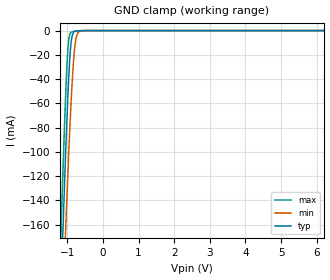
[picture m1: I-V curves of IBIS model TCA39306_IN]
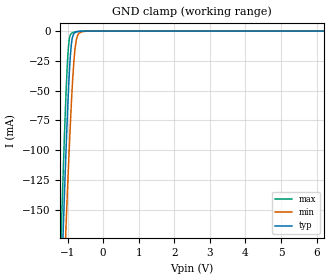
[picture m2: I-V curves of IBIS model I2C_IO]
|Texas Instruments Incorporated
| Low voltage FM+ I2C bus and SMBus voltage translator
| TCA39306
| Voltage Range : 0.9V-5.5V
| Package-type: DCU / DCT / DTM
| #pins/pkg drawing : 8-pin DCU /  8-pin DCT / 8-pin DTM
[IBIS Ver] 4.1
[File name] tca39306_5p0.ibs
[File Rev] 1.0
[Date] 07/01/2021
[Source]
| Texas Instruments Incorporated.
| 12500 TI Blvd
| Dallas, TX -75243
[Notes] Revision History:
| Rev 1.0: 07/01/2021
| - Initial version of the model
| - Model generated from simulations in SPECTRE
| - C_comp although listed in numerical order of value are
| obtained from varying PVT conditions. For PVT conditions for
| each specific value refer the buffer description under
| respective [Model]. IBIS model user is responsible for using
| appropriate C_comp to simulate for Signal Integrity.
| - Warnings regarding combined Non-monotonicity of various models have been
| reviewed and considered minor and can be ignored.
[Disclaimer]
| This model is designed as an aid for customers of Texas Instruments.
| TI and its licensors and suppliers make no warranties, either expressed
| or implied, with respect to this model, including the warranties of
| merchantability or fitness for a particular purpose. The model is
| provided solely on an "as is" basis. The entire risk as to its quality
| and performance is with the customer.
| This model is subject to change without notice. Texas Instruments
| Incorporated is not responsible for updating this model.
[Copyright]
(C) Copyright 2019 Texas Instruments Incorporated. All rights reserved.
| Component1 TCA39306DCU 8-PIN TSSOP
[Component] TCA39306_DCU
[Manufacturer] Texas Instruments Incorporated
[Package] |DCU 8-pin TSSOP
| variable typ   min   max
R_pkg 1.400e-02   1.300e-02   1.500e-02
L_pkg 1.289e-09   1.025e-09   2.014e-09
C_pkg 1.360e-13   6.600e-14   2.940e-13
[Pin]   signal_name   model_name   R_pin   L_pin   C_pin
1   GND   GND   1.400e-02   1.387e-09   1.760e-13
2   VREF1   I2C_IO   1.300e-02   1.026e-09   6.600e-14
3   SCL1   I2C_IO   1.300e-02   1.032e-09   6.700e-14
4   SDA1   I2C_IO   1.500e-02   2.014e-09   2.940e-13
5   SDA2   I2C_IO   1.400e-02   1.412e-09   1.780e-13
6   SCL2   I2C_IO   1.300e-02   1.030e-09   6.600e-14
7   VREF2   I2C_IO   1.300e-02   1.025e-09   6.600e-14
8   EN   TCA39306_IN   1.400e-02   1.386e-09   1.760e-13
[Series Pin Mapping]   pin_2   model_name   function_table_group
2   7   I2C_IO_S   1
3   6   I2C_IO_S   1
4   5   I2C_IO_S   1
[Series Switch Groups]
| Function Group States
On  1 /
Off 1 /
| Component2 TCA39306DCT 8-PIN TSSOP
[Component] TCA39306_DCT
[Manufacturer] Texas Instruments Incorporated
[Package] |DCU 8-pin TSSOP
| variable typ   min   max
R_pkg   2.900e-02   2.800e-02   3.100e-02
L_pkg   1.796e-09   1.666e-09   1.924e-09
C_pkg   1.090e-13   8.300e-14   1.360e-13
[Pin]   signal_name   model_name   R_pin   L_pin   C_pin
1   GND   GND   1.400e-02   1.387e-09   1.760e-13
2   VREF1   I2C_IO   1.300e-02   1.026e-09   6.600e-14
3   SCL1   I2C_IO   1.300e-02   1.032e-09   6.700e-14
4   SDA1   I2C_IO   1.500e-02   2.014e-09   2.940e-13
5   SDA2   I2C_IO   1.400e-02   1.412e-09   1.780e-13
6   SCL2   I2C_IO   1.300e-02   1.030e-09   6.600e-14
7   VREF2   I2C_IO   1.300e-02   1.025e-09   6.600e-14
8   EN   TCA39306_IN   1.400e-02   1.386e-09   1.760e-13
[Series Pin Mapping]   pin_2   model_name   function_table_group
2   7   I2C_IO_S   1
3   6   I2C_IO_S   1
4   5   I2C_IO_S   1
[Series Switch Groups]
| Function Group States
On 1 /
Off 1 /
| Component3 TCA39306DTM 8-PIN X2SON
[Component] TCA39306_DTM
[Manufacturer] Texas Instruments Incorporated
[Package] |DTM 8-pin X2SON
| variable typ   min   max
R_pkg   2.900e-02   2.800e-02   3.100e-02
L_pkg   1.796e-09   1.666e-09   1.924e-09
C_pkg   1.090e-13   8.300e-14   1.360e-13
[Pin]   signal_name   model_name   R_pin   L_pin   C_pin
1   GND   GND   3.000e-02   2.890e-10   7.058e-14
2   VREF1   I2C_IO   3.089e-02   2.672e-10   2.985e-13
3   SCL1   I2C_IO   3.203e-02   2.900e-10   .0654e-14
4   SDA1   I2C_IO   4.000e-02   4.124e-10   7.674e-13
5   SDA2   I2C_IO   3.190e-02   2.849e-10   1.780e-13
6   SCL2   I2C_IO   1.300e-02   2.664e-10   2.993e-13
7   VREF2   I2C_IO   3.206e-02   2.872e-10   6.541e-14
8   EN   TCA39306_IN   3.100e-02   2.839e-10   7.674e-13
[Series Pin Mapping]   pin_2   model_name   function_table_group
2   7   I2C_IO_S   1
3   6   I2C_IO_S   1
4   5   I2C_IO_S   1
[Series Switch Groups]
| Function Group States
On 1 /
Off 1 /
| I2C_IO_S
[Model]   I2C_IO_S
Model_type  Series_switch
| variable   typ   min   max
C_comp   2.6pF   2.2pF   3.5pF
[Temperature Range]   27   125   -40
[Voltage range]   5   4.5   5.5
[On]
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[Off]
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| Models and submodels in the file (3): TCA39306_IN (Input), I2C_IO_S (Series_switch), I2C_IO (Terminator)
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| TCA39306_IN
[Model]   TCA39306_IN
Model_type   Input
Vinl=1.5
Vinh=3.5
|   typ   min   max
C_comp   11pF   9.4pF   13pF
[Voltage Range]   5   4.5   5.5
[Temperature Range]   27   125   -40
[Power Clamp Reference]   5   4.5   5.5
[GND Clamp Reference]   0   0   0
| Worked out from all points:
|   GND clamp passes 1 mA (typ) near -0.81 V on its own axis
[GND Clamp]
|   Voltage   I(typ)   I(min)   I(max)
-5V       -4.053A    -3.648A    -4.173A
-1.175V   -212.7mA   -265.8mA   -165.2mA
-1.115V   -159.2mA   -217.9mA   -110.3mA
-1.04V    -96.32mA   -159.9mA   -48.86mA
-995mV    -62.32mA   -126.7mA   -20.83mA
-965mV    -42.37mA   -105.5mA   -9.183mA
-920mV    -18.97mA   -75.54mA   -2.431mA
-875mV    -6.08mA    -48.91mA   -1.124mA
-800mV    -796.4uA   -16.51mA   -628.6uA
-755mV    -348.1uA   -6.535mA   -457.5uA
-620mV    -55.53uA   -280.6uA   -114.4uA
10V       0A         0A         0A
| I2C_IO
[Model]   I2C_IO
Model_type  Terminator
|   typ   min   max
C_comp   2.6pF   2.2pF   3.5pF
[Voltage Range]   5   4.5   5.5
[Temperature Range]   27   125   -40
[Power Clamp Reference]   5   4.5   5.5
[GND Clamp Reference]   0   0   0
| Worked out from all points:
|   GND clamp passes 1 mA (typ) near -0.78 V on its own axis
[GND Clamp]
|   Voltage   I(typ)   I(min)   I(max)
-5V       -4.07A     -3.665A    -4.191A
-1.175V   -214.8mA   -268.3mA   -166.9mA
-1.13V    -174.3mA   -232.1mA   -125.2mA
-1.115V   -161.1mA   -220.2mA   -111.8mA
-1.055V   -110mA     -173.4mA   -61.36mA
-1.04V    -97.87mA   -162mA     -50.06mA
-980mV    -53.36mA   -117.8mA   -15.17mA
-920mV    -20.13mA   -77.21mA   -3.116mA
-830mV    -2.45mA    -28.64mA   -959.4uA
-725mV    -481.3uA   -4.237mA   -364.8uA
-500mV    -6.727uA   -150.8uA   -12.47uA
10V       0A         0A         0A
